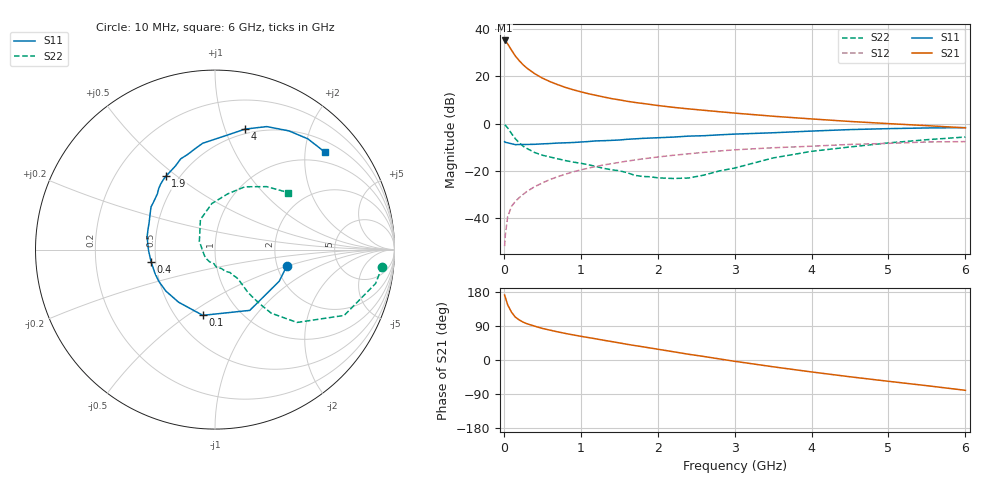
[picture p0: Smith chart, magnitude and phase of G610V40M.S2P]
! SIEMENS Small Signal Semiconductors
! BFG193
! Si NPN RF Bipolar Junction Transistor in SOT223
! VCE = 10 V  IC = 40 mA
! Common Emitter S-Parameters:  August  1996
# GHz  S  MA  R  50
!  f  S11  S21  S12  S22
! GHz  MAG  ANG  MAG  ANG  MAG  ANG  MAG  ANG
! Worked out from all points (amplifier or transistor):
!   36 points, 10 MHz to 6 GHz, reference 50 ohm
!   highest |S21| = 35.3 dB at 10 MHz (marker M1)
!   |S21| within 3 dB of that: start of sweep to 78.84 MHz
!   unconditionally stable (mu >= 1): 554.3 MHz to 2.534 GHz
!   at 250 MHz: K = 0.86, MSG = 27.5 dB, |S12| = -30.1 dB
!   at 1.4 GHz: K = 1.04, MAG = 12.6 dB, |S12| = -17.0 dB
!   at 6 GHz: K = 0.89, MSG = 2.9 dB, |S12| = -7.7 dB
!   S11 on the Smith chart (normalised r, x): 10 MHz: 2.26, -0.49; 100 MHz: 0.68, -0.57; 400 MHz: 0.47, -0.07; 1.9 GHz: 0.42, +0.46; 4 GHz: 0.46, +1.17; 6 GHz: 0.74, +2.44
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0.01  0.4106 -12.8  57.88 171.4  0.0025 85.6  0.9363 -5.8
0.02  0.3988 -26.3  56.28 164.8  0.0044 80.3  0.9147 -11.9
0.05  0.3902 -60.2  48.85 145.5  0.0106 71.6  0.8079 -27.0
0.1  0.3725 -100.5  36.01 126.0  0.0175 65.3  0.6113 -41.6
0.15  0.3565 -124.7  27.03 113.1  0.0223 63.4  0.4732 -48.5
0.2  0.3582 -139.9  21.54 105.7  0.0268 65.1  0.3913 -50.5
0.25  0.3594 -150.6  17.68 100.0  0.0313 64.5  0.3306 -51.8
0.3  0.3597 -158.3  14.97 95.7  0.0362 66.1  0.2956 -52.4
0.4  0.3625 -169.3  11.44 89.4  0.0457 66.6  0.2431 -52.1
0.5  0.3701 -179.0  9.216 83.4  0.0548 66.1  0.2128 -51.8
0.6  0.376 175.0  7.75 78.8  0.0649 65.5  0.1949 -52.5
0.7  0.3849 169.0  6.681 74.3  0.0744 64.5  0.1788 -54.3
0.9  0.3957 158.3  5.215 66.3  0.0944 61.4  0.1523 -56.8
1.1  0.4148 150.4  4.291 59.2  0.1133 58.1  0.1337 -64.6
1.4  0.4394 138.9  3.381 48.7  0.1405 52.1  0.1045 -77.0
1.9  0.4916 123.9  2.543 31.8  0.1858 41.7  0.0743 -114.8
2.2  0.5154 115.3  2.208 21.9  0.2117 34.6  0.0682 -146.4
3.5  0.6369 84.8  1.428 -17.9  0.3061 3.9  0.186 115.9
4  0.6919 76.0  1.252 -31.5  0.3301 -5.8  0.2573 93.9
4.5  0.7435 67.2  1.106 -44.3  0.3604 -15.9  0.3183 77.2
5.5  0.8053 50.0  0.901 -67.8  0.4063 -39.0  0.4538 50.6
6  0.8186 41.5  0.81 -80.0  0.4137 -52.3  0.5172 37.9
